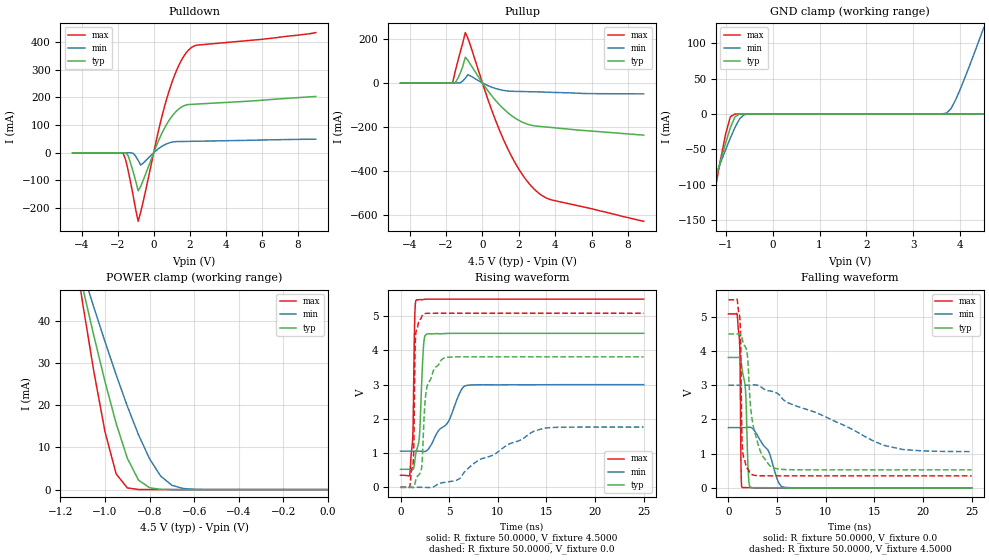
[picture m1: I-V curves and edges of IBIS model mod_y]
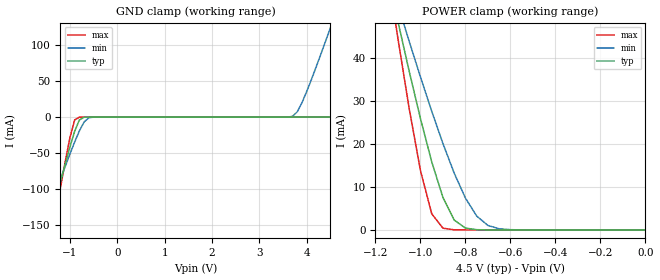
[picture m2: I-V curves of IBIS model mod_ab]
| IBIS file 54ac02.ibs created by s2ibis3 verion 1.1
| North Carolina State University, ERL, 2006
[IBIS ver]  4.0
[File name] 54ac02_4v5_rev1.ibs
[File Rev]  1.0
[Date]   23 March 2012
[Source]   CAD & Design Services (Catania) - STMicroelectronics
[Notes]
  (Note1) This IBIS model is the model of the product with package
   (Flat14 package elements);
  (Note2) This IBIS model is extracted with nominal 4.5V power supply
   (min:3.0V, typ:4.5V, max:5.5V);
  (Note3) This model has few Warnings about the non-monotonicity
   of I-V curves, but they are not indicative of problems
   inside the model;
[Copyright] (c) 2012 STMicroelectronics
|   Component 54AC02
[Component] 54AC02
[Manufacturer] STMicroelectronics
[Package]
| variable   typ   min   max
R_pkg   0.0   0.0   0.0
L_pkg   0.0H   0.0H   0.0H
C_pkg   0.0F   0.0F   0.0F
[Pin]   signal_name   model_name   R_pin   L_pin   C_pin
1   1Y   mod_y   141.0m   4.31nH   1.01pF
2   1A   mod_ab   108.1m   3.05nH   1.04pF
3   1B   mod_ab   90.5m   2.36nH   0.8pF
4   2Y   mod_y   79.7m   1.96nH   0.8pF
5   2A   mod_ab   86.2m   2.16nH   0.8pF
6   2B   mod_ab   101.7m   2.85nH   1.04pF
7   GND   GND   111.0m   3.51nH   1.01pF
8   3A   mod_ab   141.0m   4.31nH   1.01pF
9   3B   mod_ab   112.4m   3.25nH   1.04pF
10   3Y   mod_y   90.5m   2.36nH   0.8pF
11   4A   mod_ab   81.9m   2.06nH   0.8pF
12   4B   mod_ab   84.0m   2.16nH   0.8pF
13   4Y   mod_y   101.7m   2.85nH   1.04pF
14   VCC   POWER   111.0m   3.51nH   1.01pF
| Models and submodels in the file (2): mod_y (I/O), mod_ab (Input)
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|   Model mod_y
[Model]   mod_y
Model_type I/O
Polarity   Inverting
Vinl   =   0.90V
Vinh   =   2.10V
Vmeas  =   2.25V
Cref   =   50pF
Rref   =   500
C_comp   3.063pF   NA   NA
[Temperature Range]   25.0000   0.1250k   -55.0000
[Voltage Range]   4.5000V   3.0000V   5.5000V
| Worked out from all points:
|   slope of the pulldown table from 0 to 0.675 V, typ, clamps not added: 6.92 ohm
|   slope of the pullup table from 0 to 0.675 V, typ, clamps not added: 8.98 ohm
|   GND clamp passes 1 mA (typ) near -0.72 V on its own axis
|   POWER clamp passes 1 mA (typ) near -0.82 V on its own axis
|   rising waveform, R_fixture 50.0000, V_fixture 4.5000: 20-80 % time 403ps typ, 2.37ns min, 185ps max; typ from 0.527 V to 4.5 V
|   rising waveform, R_fixture 50.0000, V_fixture 0.0: 20-80 % time 629ps typ, 6.19ns min, 152ps max; typ from 0 V to 3.81 V
|   falling waveform, R_fixture 50.0000, V_fixture 0.0: 20-80 % time 302ps typ, 1.67ns min, 108ps max; typ from 3.81 V to 0 V
|   falling waveform, R_fixture 50.0000, V_fixture 4.5000: 20-80 % time 997ps typ, 8.86ns min, 154ps max; typ from 4.5 V to 0.527 V
[Pulldown]
|Voltage   I(typ)   I(min)   I(max)
-4.5V     0A         0A         0A
-1.7V     0A         0A         0A
-1.42V    -9.78mA    0A         -62.62mA
-1.14V    -67.56mA   -1.748mA   -153.5mA
-860mV    -137.4mA   -27.48mA   -247.5mA
-720mV    -121.7mA   -44.44mA   -214.9mA
260mV     42.23mA    14.38mA    77.67mA
680mV     98.1mA     30.97mA    184.9mA
1.38V     157.3mA    40.54mA    313.4mA
1.94V     174.3mA    41.15mA    371.1mA
2.36V     175.8mA    41.61mA    388.1mA
9V        203.2mA    49.15mA    434.1mA
[Pullup]
|Voltage   I(typ)   I(min)   I(max)
-4.5V     0A         0A         0A
-1.64V    0A         0A         0A
-1.5V     0A         0A         51.02mA
-1.36V    19.22mA    0A         96.83mA
-940mV    117mA      21.37mA    229.5mA
-800mV    103.6mA    37.66mA    203.9mA
320mV     -37.87mA   -12.88mA   -79.72mA
1.02V     -106.7mA   -31.88mA   -231.8mA
1.86V     -163.8mA   -38.63mA   -373.8mA
2.7V      -193.2mA   -40.32mA   -471.7mA
3.68V     -202.4mA   -42.69mA   -530.2mA
8.86V     -238mA     -49.97mA   -630.8mA
[GND_clamp]
|Voltage   I(typ)   I(min)   I(max)
-4.5V     -947.8mA   -697.3mA   -1.362A
-1.7V     -215.2mA   -175mA     -283.7mA
-1.6V     -189.5mA   -156.7mA   -245.8mA
-1.5V     -164mA     -138.6mA   -208.1mA
-1.4V     -138.6mA   -120.5mA   -170.6mA
-1V       -40.81mA   -50.28mA   -28.18mA
-900mV    -19.37mA   -33.88mA   -3.841mA
-800mV    -3.851mA   -18.75mA   -31.64uA
-500mV    -57.51nA   -52.83uA   -10.23pA
3.7V      2.9pA      1.031mA    1.9pA
3.9V      3.3pA      19.76mA    2.3pA
4.5V      4.5pA      121.8mA    3.5pA
[POWER_clamp]
|Voltage   I(typ)   I(min)   I(max)
-4.5V     929.4mA    679.8mA    1.342A
-1.15V    59.57mA    59.97mA    61.08mA
-1.1V     47.81mA    51.47mA    44.01mA
-1.05V    36.4mA     43.14mA    27.9mA
-1V       25.55mA    35.01mA    13.66mA
-950mV    15.63mA    27.17mA    3.721mA
-900mV    7.436mA    19.76mA    409.3uA
-850mV    2.267mA    13mA       30.16uA
-750mV    63.91uA    3.182mA    148.2nA
-700mV    9.201uA    1.031mA    10.38nA
-600mV    187.9nA    64.84uA    57.46pA
0V        4.5pA      41.65pA    5.5pA
[Ramp]
| variable   typ   min   max
dV/dt_r  2.2880/0.7396n   1.0571/6.1963n   3.0521/0.2424n
dV/dt_f  2.3840/1.0323n   1.1659/8.8843n   3.0889/0.2859n
R_load = 50.0000
[Rising Waveform]
R_fixture= 50.0000
V_fixture= 4.5000
V_fixture_min= 3.0000
V_fixture_max= 5.5000
|time   V(typ)   V(min)   V(max)
0s        526.6mV    1.057V     351.6mV
975ps     526.7mV    1.057V     421.5mV
1.275ns   522.7mV    1.057V     1.566V
1.45ns    724.9mV    1.057V     4.821V
1.625ns   1.06V      1.057V     5.478V
1.975ns   1.622V     1.056V     5.486V
2.375ns   4.168V     1.047V     5.49V
2.675ns   4.479V     1.065V     5.499V
6.625ns   4.5V       2.964V     5.5V
25ns      4.5V       3V         5.5V
[Rising Waveform]
R_fixture= 50.0000
V_fixture= 0.0
V_fixture_min= 0.0
V_fixture_max= 0.0
|time   V(typ)   V(min)   V(max)
0s        0V         0V         0V
950ps     -59.74uV   1.134uV    -6.455mV
1.3ns     -16.21mV   -9.099uV   716.8mV
1.55ns    191.2mV    -30.4uV    4.44V
2.15ns    537.3mV    478.1uV    4.969V
2.35ns    1.566V     -164.9uV   5.058V
2.75ns    2.973V     -5.046mV   5.085V
4.45ns    3.777V     141.5mV    5.087V
14.83ns   3.814V     1.731V     5.087V
25ns      3.814V     1.762V     5.087V
[Falling Waveform]
R_fixture= 50.0000
V_fixture= 0.0
V_fixture_min= 0.0
V_fixture_max= 0.0
|time   V(typ)   V(min)   V(max)
0s        3.814V     1.762V     5.087V
1.125ns   3.824V     1.762V     4.37V
1.2ns     3.811V     1.762V     3.572V
1.3ns     3.698V     1.761V     482.9mV
1.425ns   3.427V     1.761V     12.12mV
1.75ns    2.875V     1.762V     8.281mV
2.05ns    388.7mV    1.77V      6.923mV
2.25ns    22.94mV    1.771V     6.271mV
5.45ns    705.2uV    39.7mV     -417.4nV
25ns      -1.392uV   11.39uV    -771.1nV
[Falling Waveform]
R_fixture= 50.0000
V_fixture= 4.5000
V_fixture_min= 3.0000
V_fixture_max= 5.5000
|time   V(typ)   V(min)   V(max)
0s        4.5V       3V         5.5V
1.15ns    4.518V     3V         5.033V
1.25ns    4.508V     3V         4.413V
1.375ns   4.404V     3V         1.621V
1.45ns    4.313V     3V         1.099V
1.95ns    3.872V     2.999V     562.2mV
2.35ns    2.181V     3.005V     400mV
4.8ns     571.3mV    2.794V     351.6mV
15.97ns   526.6mV    1.244V     351.6mV
25ns      526.6mV    1.059V     351.6mV
|   Model mod_ab
[Model]   mod_ab
Model_type Input
Vinl   =   0.90V
Vinh   =   2.10V
C_comp   0.532pF   NA   NA
[Temperature Range]  25.0000   0.1250k   -55.0000
[Voltage Range]   4.5000V   3.0000V   5.5000V
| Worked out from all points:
|   GND clamp passes 1 mA (typ) near -0.72 V on its own axis
|   POWER clamp passes 1 mA (typ) near -0.82 V on its own axis
[GND_clamp]
|Voltage   I(typ)   I(min)   I(max)
-4.5V     -962.5mA   -710.6mA   -1.378A
-1.7V     -218.5mA   -178.3mA   -287.1mA
-1.6V     -192.5mA   -159.7mA   -248.8mA
-1.5V     -166.5mA   -141.2mA   -210.6mA
-1.4V     -140.8mA   -122.8mA   -172.7mA
-1V       -41.47mA   -51.24mA   -28.54mA
-900mV    -19.68mA   -34.52mA   -3.902mA
-800mV    -3.919mA   -19.11mA   -32.25uA
-500mV    -58.62nA   -53.84uA   -16.8pA
3.7V      5.8pA      1.051mA    3.8pA
3.9V      6.6pA      20.13mA    4.6pA
4.5V      9.001pA    124.1mA    7pA
[POWER_clamp]
|Voltage   I(typ)   I(min)   I(max)
-4.5V     943.9mA    692.8mA    1.358A
-1.15V    60.51mA    61.11mA    61.84mA
-1.1V     48.57mA    52.46mA    44.58mA
-1.05V    36.98mA    43.96mA    28.26mA
-1V       25.96mA    35.67mA    13.85mA
-950mV    15.89mA    27.69mA    3.78mA
-900mV    7.563mA    20.13mA    416.9uA
-850mV    2.308mA    13.24mA    30.74uA
-750mV    65.13uA    3.242mA    151.1nA
-700mV    9.377uA    1.051mA    10.58nA
-600mV    191.5nA    66.07uA    65.13pA
0V        9.001pA    45.39pA    11pA
